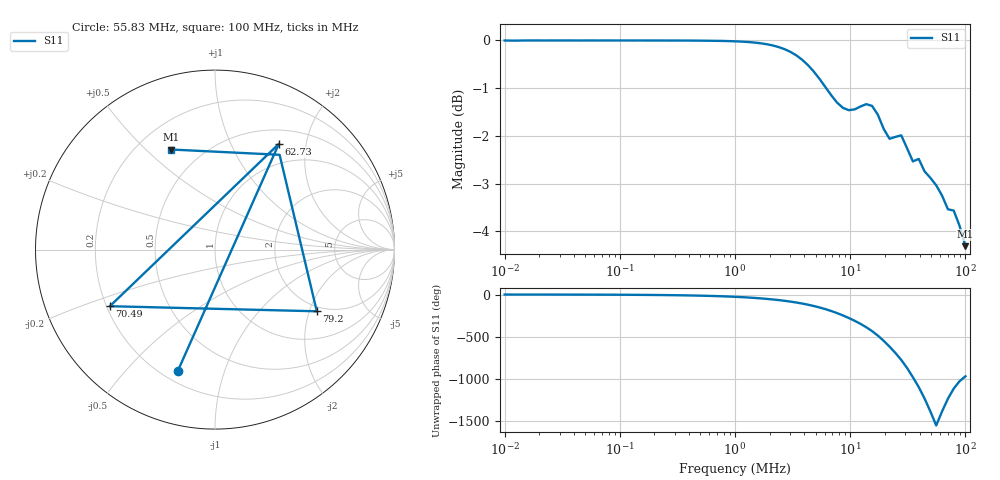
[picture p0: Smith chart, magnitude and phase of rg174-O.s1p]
! ListType=Log
!!RG174 24.9f Open
# MHz S RI R 50
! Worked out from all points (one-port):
!   80 points, 10 kHz to 100 MHz, reference 50 ohm
!   lowest |S11| = -4.3 dB at 100 MHz (marker M1), VSWR 4.11, Z = 16.9 + j30 ohm
!   |S11| at or under -10 dB: nowhere
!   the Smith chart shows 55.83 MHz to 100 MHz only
!   S11 on the Smith chart (normalised r, x): 55.83 MHz: 0.26, -0.71; 62.73 MHz: 0.69, +1.54; 70.49 MHz: 0.21, -0.24; 79.2 MHz: 1.83, -2.25; 100 MHz: 0.34, +0.60
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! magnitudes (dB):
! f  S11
! 10 kHz  0.0
! 32.09 kHz  0.0
! 103 kHz  0.0
! 330.4 kHz  0.0
! 1.06 MHz  0.0
! 2.134 MHz  -0.1
! 2.694 MHz  -0.2
! 3.401 MHz  -0.3
! 4.826 MHz  -0.7
! 7.693 MHz  -1.3
! 8.644 MHz  -1.4
! 9.713 MHz  -1.5
! 10.91 MHz  -1.4
! 13.78 MHz  -1.3
! 15.48 MHz  -1.4
! 17.4 MHz  -1.6
! 19.55 MHz  -1.9
! 21.97 MHz  -2.1
! 27.74 MHz  -2.0
! 35.02 MHz  -2.5
! 39.35 MHz  -2.5
! 44.21 MHz  -2.7
! 55.83 MHz  -3.0
! 62.73 MHz  -3.3
! 70.49 MHz  -3.5
! 79.2 MHz  -3.6
! 89 MHz  -3.9
! 100 MHz  -4.3
